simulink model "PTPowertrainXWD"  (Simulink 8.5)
settings: Solver=ode45  StartTime=0.0  StopTime=inf  RelTol=1e-3
libraries: CarMaker4SL x9, simulink x1
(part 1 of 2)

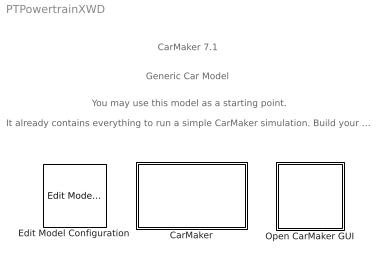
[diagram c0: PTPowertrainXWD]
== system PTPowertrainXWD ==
  note: Generic Car Model
  note: You may use this model as a starting point.
  note: It already contains everything to run a simple CarMaker simulation. Build your Simulink model around it.
  note: CarMaker 7.1
  CarMaker : Subsystem  TreatAsAtomicUnit=on
  Edit Model Configuration : CarMaker4SL/Edit Model Configuration
  Open CarMaker GUI : Subsystem  LoadFcn=if ~length(which('cmself')), cmenv; end

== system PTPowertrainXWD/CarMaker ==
  CM_FIRST : Subsystem
  CM_LAST : Subsystem
  DrivMan : Subsystem
  Ground : Ground
  IPG Vehicle : Subsystem  TreatAsAtomicUnit=on
  Terminator : Terminator
  VehicleControl : Subsystem
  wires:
  DrivMan/2(DrivMan.Out) -> VehicleControl/2(DrivMan.In)
  DrivMan/1(Sync_Out) -> VehicleControl/1(Sync_In)
  CM_FIRST/2(Env.Misc) -> DrivMan/2(Env.Misc)
  CM_FIRST/1(Sync_Out) -> DrivMan/1(Sync_In)
  CM_LAST/1(Sync_Out) -> Terminator/1
  Ground/1 -> CM_FIRST/1(Sync_In)
  IPG Vehicle/1(Sync_Out) -> CM_LAST/1(Sync_In)
  VehicleControl/1(Sync_Out) -> IPG Vehicle/1(Sync_In)
  VehicleControl/3(VhclCtrl.Steering) -> IPG Vehicle/3(VhclCtrl.Steering)
  VehicleControl/4(Vhcl.Wheel.In) -> IPG Vehicle/4(Vhcl.Wheel.In)
  VehicleControl/5(Vhcl.Misc) -> IPG Vehicle/5(Vhcl.Misc)
  VehicleControl/6(VhclCtrl.Brake) -> IPG Vehicle/6(VhclCtrl.Brake)
  VehicleControl/7(VhclCtrl.PT) -> IPG Vehicle/7(VhclCtrl.PT)
  VehicleControl/2(Vhcl.Model.Source) -> IPG Vehicle/2(Vhcl.Model.Source)

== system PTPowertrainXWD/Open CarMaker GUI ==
  S-Function : S-Function  FunctionName=cm_gui

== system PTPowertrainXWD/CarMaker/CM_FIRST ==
  Sync_In : Inport
  BusCreator1 : BusCreator  Inputs=8
  BusCreator2 : BusCreator  Inputs=6
  Demux1 : Demux  Outputs=14
  Environment : S-Function  FunctionName=CM_Sfun  Parameters='Environment'
  IoIn : S-Function  FunctionName=CM_Sfun  Parameters='IoIn'
  Terminator : Terminator
  Sync_Out : Outport
  Env.Misc : Outport  Port=2
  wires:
  BusCreator2/1 -> Terminator/1  "IF Environment (in)"
  BusCreator1/1 -> Env.Misc/1
  Demux1/14 -> BusCreator2/6  "Env sRoad"
  Demux1/13 -> BusCreator2/5  "Env PoI_GCS Elev"
  Demux1/12 -> BusCreator2/4  "Env PoI_GCS Lat"
  Demux1/11 -> BusCreator2/3  "Env PoI_GCS Long"
  Demux1/10 -> BusCreator2/2  "Env Time"
  Demux1/9 -> BusCreator2/1  "Env yDay"
  Demux1/8 -> BusCreator1/8  "Env WindVel_tot z"
  Demux1/7 -> BusCreator1/7  "Env WindVel_tot y"
  Demux1/6 -> BusCreator1/6  "Env WindVel_tot x"
  Demux1/5 -> BusCreator1/5  "Env SolarRadiation"
  Demux1/4 -> BusCreator1/4  "Env AirHumidity"
  Demux1/3 -> BusCreator1/3  "Env AirPressure"
  Demux1/2 -> BusCreator1/2  "Env AirDensity"
  Demux1/1 -> BusCreator1/1  "Env Temperature"
  Environment/2 -> Demux1/1
  Environment/1 -> Sync_Out/1
  IoIn/1 -> Environment/1
  Sync_In/1 -> IoIn/1

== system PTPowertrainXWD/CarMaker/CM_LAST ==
  Sync_In : Inport
  CM_User : S-Function  FunctionName=CM_Sfun  Parameters='CM_User'
  IoOut : S-Function  FunctionName=CM_Sfun  Parameters='IoOut'
  Sync_Out : Outport
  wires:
  IoOut/1 -> Sync_Out/1
  CM_User/1 -> IoOut/1
  Sync_In/1 -> CM_User/1

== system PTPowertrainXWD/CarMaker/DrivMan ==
  note: There's rarely a reason to override DrivMan signals. Use the VehicleControl interface for this purpose.
  Sync_In : Inport
  Env.Misc : Inport  Port=2
  BusCreator : BusCreator  Inputs=17
  Demux : Demux  Outputs=17
  DrivMan : S-Function  FunctionName=CM_Sfun  Parameters='DrivMan'
  Sync_Out : Outport
  DrivMan.Out : Outport  Port=2
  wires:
  Demux/17 -> BusCreator/17  "DrivMan Steering Trq"
  Demux/16 -> BusCreator/16  "DrivMan Steering AngAcc"
  Demux/15 -> BusCreator/15  "DrivMan Steering AngVel"
  Demux/14 -> BusCreator/14  "DrivMan Steering Ang"
  Demux/13 -> BusCreator/13  "DrivMan Gas"
  Demux/12 -> BusCreator/12  "DrivMan Clutch"
  Demux/11 -> BusCreator/11  "DrivMan BrakePark"
  Demux/10 -> BusCreator/10  "DrivMan Brake"
  Demux/9 -> BusCreator/9  "DrivMan GearNo"
  Demux/8 -> BusCreator/8  "DrivMan SelectorCtrl"
  Demux/7 -> BusCreator/7  "DrivMan UserSignal4"
  Demux/6 -> BusCreator/6  "DrivMan UserSignal3"
  Demux/5 -> BusCreator/5  "DrivMan UserSignal2"
  Demux/4 -> BusCreator/4  "DrivMan UserSignal1"
  Demux/3 -> BusCreator/3  "DrivMan UserSignal0"
  Demux/2 -> BusCreator/2  "DrivMan Key"
  Demux/1 -> BusCreator/1  "DrivMan SST"
  Env.Misc/1 -> DrivMan/2
  Sync_In/1 -> DrivMan/1
  DrivMan/1 -> Sync_Out/1
  BusCreator/1 -> DrivMan.Out/1
  DrivMan/2 -> Demux/1

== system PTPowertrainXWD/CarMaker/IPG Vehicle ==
  Sync_In : Inport
  Vhcl.Model.Source : Inport  Port=2
  VhclCtrl.Steering : Inport  Port=3
  Vhcl.Wheel.In : Inport  Port=4
  Vhcl.Misc : Inport  Port=5
  VhclCtrl.Brake : Inport  Port=6
  VhclCtrl.PT : Inport  Port=7
  Brake : Subsystem
  CarAndTrailer : Subsystem
  PowerTrain : Subsystem
  Stop Simulation : Stop
  VehicleSource_BuiltIn : simulink/Logic and Bit Operations/Compare To Constant  relop=~=  const=1  OutDataTypeStr=boolean  ZeroCross=off
  Sync_Out : Outport
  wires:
  VhclCtrl.PT/1 -> PowerTrain/3(VhclCtrl.PT)
  Brake/1(Sync_Out) -> PowerTrain/1(Sync_In)
  CarAndTrailer/1(Sync_Out) -> Brake/1(Sync_In)
  CarAndTrailer/2(Brake.IF.In) -> Brake/2(Brake.IF.In)
  VhclCtrl.Brake/1 -> Brake/3(VhclCtrl.Brake)
  PowerTrain/1(Sync_Out) -> Sync_Out/1
  Vhcl.Misc/1 -> CarAndTrailer/4(Vhcl.Misc)
  Vhcl.Wheel.In/1 -> CarAndTrailer/3(Vhcl.Wheel.In)
  VhclCtrl.Steering/1 -> CarAndTrailer/2(VhclCtrl.Steering)
  Sync_In/1 -> CarAndTrailer/1(Sync_In)
  Vhcl.Model.Source/1 -> VehicleSource_BuiltIn/1
  VehicleSource_BuiltIn/1 -> Stop Simulation/1
  Brake/2(Vhcl.Wheel.PT) -> PowerTrain/2(Vhcl.Wheel.PT)

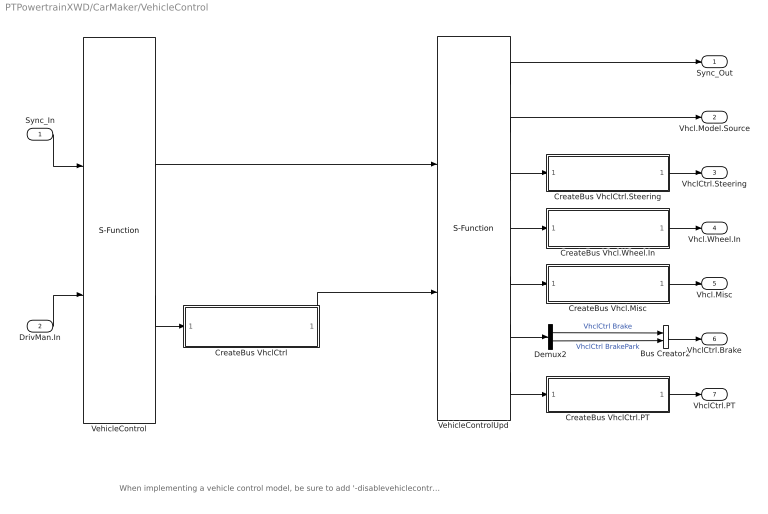
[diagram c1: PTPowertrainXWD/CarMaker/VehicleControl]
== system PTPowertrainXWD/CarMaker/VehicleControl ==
  note: When implementing a vehicle control model, be sure to add '-disablevehiclecontrol' to the command line arguments in the CarMaker Model Configuration block. Otherwise your model will possibly not see the original DrivMan signals on its inputs, but those of a currently activated C-coded vehicle control model instead.
  Sync_In : Inport
  DrivMan.In : Inport  Port=2
  Bus Creator2 : BusCreator  Inputs=2
  CreateBus Vhcl.Misc : Subsystem
  CreateBus Vhcl.Wheel.In : Subsystem
  CreateBus VhclCtrl : Subsystem
  CreateBus VhclCtrl.PT : Subsystem
  CreateBus VhclCtrl.Steering : Subsystem
  Demux2 : Demux  Outputs=2
  VehicleControl : S-Function  FunctionName=CM_Sfun  Parameters='VehicleControl'
  VehicleControlUpd : S-Function  FunctionName=CM_Sfun  Parameters='VehicleControlUpd'
  Sync_Out : Outport
  Vhcl.Model.Source : Outport  Port=2
  VhclCtrl.Steering : Outport  Port=3
  Vhcl.Wheel.In : Outport  Port=4
  Vhcl.Misc : Outport  Port=5
  VhclCtrl.Brake : Outport  Port=6
  VhclCtrl.PT : Outport  Port=7
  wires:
  CreateBus VhclCtrl/1(Out) -> VehicleControlUpd/2
  VehicleControl/2 -> CreateBus VhclCtrl/1(In)
  VehicleControlUpd/2 -> Vhcl.Model.Source/1
  VehicleControlUpd/4 -> CreateBus Vhcl.Wheel.In/1(In1)
  VehicleControlUpd/5 -> CreateBus Vhcl.Misc/1(In1)
  VehicleControlUpd/6 -> Demux2/1
  VehicleControlUpd/7 -> CreateBus VhclCtrl.PT/1(In1)
  VehicleControlUpd/3 -> CreateBus VhclCtrl.Steering/1(In1)
  CreateBus Vhcl.Misc/1(Out1) -> Vhcl.Misc/1
  CreateBus Vhcl.Wheel.In/1(Out1) -> Vhcl.Wheel.In/1
  DrivMan.In/1 -> VehicleControl/2
  VehicleControl/1 -> VehicleControlUpd/1
  Sync_In/1 -> VehicleControl/1
  CreateBus VhclCtrl.PT/1(Out1) -> VhclCtrl.PT/1
  Bus Creator2/1 -> VhclCtrl.Brake/1
  CreateBus VhclCtrl.Steering/1(Out1) -> VhclCtrl.Steering/1
  VehicleControlUpd/1 -> Sync_Out/1
  Demux2/2 -> Bus Creator2/2  "VhclCtrl BrakePark"
  Demux2/1 -> Bus Creator2/1  "VhclCtrl Brake"

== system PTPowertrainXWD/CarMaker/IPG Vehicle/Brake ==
  note: When replacing the entire braking system, be sure to add '-disablebrake' to the command line arguments in the CarMaker Model Configuration block.
  Sync_In : Inport
  Brake.IF.In : Inport  Port=2
  VhclCtrl.Brake : Inport  Port=3
  Brake : S-Function  FunctionName=CM_Sfun  Parameters='Brake'
  BrakeUpd : S-Function  FunctionName=CM_Sfun  Parameters='BrakeUpd'
  BusCreator1 : BusCreator  Inputs=16
  CreateBus Vhcl.Wheel.PT : Subsystem
  Demux : Demux  Outputs=16
  Sync_Out : Outport
  Vhcl.Wheel.PT : Outport  Port=2
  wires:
  Demux/16 -> BusCreator1/16  "Brake IF Trq_DriveSrc_trg d3"
  Demux/15 -> BusCreator1/15  "Brake IF Trq_DriveSrc_trg d2"
  Demux/14 -> BusCreator1/14  "Brake IF Trq_DriveSrc_trg d1"
  Demux/13 -> BusCreator1/13  "Brake IF Trq_DriveSrc_trg d0"
  Demux/12 -> BusCreator1/12  "Brake IF Trq_Reg_trg RR"
  Demux/11 -> BusCreator1/11  "Brake IF Trq_Reg_trg RL"
  Demux/10 -> BusCreator1/10  "Brake IF Trq_Reg_trg FR"
  Demux/9 -> BusCreator1/9  "Brake IF Trq_Reg_trg FL"
  Demux/8 -> BusCreator1/8  "Brake IF Trq_PB RR"
  Demux/7 -> BusCreator1/7  "Brake IF Trq_PB RL"
  Demux/6 -> BusCreator1/6  "Brake IF Trq_PB FR"
  Demux/5 -> BusCreator1/5  "Brake IF Trq_PB FL"
  Demux/4 -> BusCreator1/4  "Brake IF Trq_WB RR"
  Demux/3 -> BusCreator1/3  "Brake IF Trq_WB RL"
  Demux/2 -> BusCreator1/2  "Brake IF Trq_WB FR"
  Demux/1 -> BusCreator1/1  "Brake IF Trq_WB FL"
  Brake/2 -> Demux/1
  BusCreator1/1 -> BrakeUpd/2
  BrakeUpd/1 -> Sync_Out/1
  Brake/1 -> BrakeUpd/1  "Sync"
  Brake.IF.In/1 -> Brake/2
  VhclCtrl.Brake/1 -> Brake/3
  Sync_In/1 -> Brake/1
  BrakeUpd/2 -> CreateBus Vhcl.Wheel.PT/1(In)
  CreateBus Vhcl.Wheel.PT/1(Out) -> Vhcl.Wheel.PT/1

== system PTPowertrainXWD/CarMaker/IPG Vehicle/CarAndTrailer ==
  Sync_In : Inport
  VhclCtrl.Steering : Inport  Port=2
  Vhcl.Wheel.In : Inport  Port=3
  Vhcl.Misc : Inport  Port=4
  CarAndTrailerUpd : Subsystem
  Forces : Subsystem
  Ground : Ground
  Kinematics : Subsystem
  Kinetics : Subsystem
  Steering : Subsystem
  Terminator : Terminator
  Terminator1 : Terminator
  Trailer : Subsystem
  Sync_Out : Outport
  Brake.IF.In : Outport  Port=2
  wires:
  Trailer/9(Car.Hitch.FrcTrq) -> CarAndTrailerUpd/9(Car.Hitch.FrcTrq)
  Trailer/8(Vhcl.Wheel.RR) -> CarAndTrailerUpd/8(Vhcl.Wheel.RR)
  Trailer/7(Vhcl.Wheel.RL) -> CarAndTrailerUpd/7(Vhcl.Wheel.RL)
  Trailer/6(Vhcl.Wheel.FR) -> CarAndTrailerUpd/6(Vhcl.Wheel.FR)
  Trailer/5(Vhcl.Wheel.FL) -> CarAndTrailerUpd/5(Vhcl.Wheel.FL)
  Trailer/4(Vhcl.PoI) -> CarAndTrailerUpd/4(Vhcl.PoI)
  Trailer/3(Vhcl.Motion) -> CarAndTrailerUpd/3(Vhcl.Motion)
  Trailer/2(Vhcl.Steering) -> CarAndTrailerUpd/2(Vhcl.Steering)
  Trailer/1(Sync_Out) -> CarAndTrailerUpd/1(Sync_In)
  CarAndTrailerUpd/2(Brake.IF.In) -> Brake.IF.In/1
  CarAndTrailerUpd/1(Sync_Out) -> Sync_Out/1
  Vhcl.Misc/1 -> Terminator1/1
  Vhcl.Wheel.In/1 -> Terminator/1
  Kinetics/6(WheelCarrier.Misc) -> Trailer/6(WheelCarrier.Misc)
  Kinetics/5(Car.Trq_T2W) -> Trailer/5(Car.Trq_T2W)
  Steering/2(Steer.IF) -> Kinematics/2(Steer.IF)
  Kinetics/4(Car.Fr1) -> Trailer/4(Car.Fr1)
  Kinetics/3(Car.Hitch) -> Trailer/3(Car.Hitch)
  Kinetics/2(Trailer.Load) -> Trailer/2(Trailer.Load)
  VhclCtrl.Steering/1 -> Steering/2(VhclCtrl.Steering)
  Sync_In/1 -> Steering/1(Sync_In)
  Steering/1(Sync_Out) -> Kinematics/1(Sync_In)
  Kinetics/1(Sync_Out) -> Trailer/1(Sync_In)
  Ground/1 -> CarAndTrailerUpd/10(Vhcl.Fr1A)
  Forces/11(FStabi) -> Kinetics/11(FStabi)
  Forces/10(FDamp) -> Kinetics/10(FDamp)
  Forces/9(FSpring) -> Kinetics/9(FSpring)
  Forces/8(TireRR_Out) -> Kinetics/8(TireRR.Out)
  Forces/7(TireRL_Out) -> Kinetics/7(TireRL.Out)
  Forces/6(TireFR_Out) -> Kinetics/6(TireFR.Out)
  Forces/5(TireFL_Out) -> Kinetics/5(TireFL.Out)
  Forces/4(Car.Load) -> Kinetics/4(Car.Load)
  Forces/2(Car.Virtual) -> Kinetics/2(Car.Virtual)
  Kinematics/6(lSpring) -> Forces/6(lSpring)
  Kinematics/7(vDamp) -> Forces/7(vDamp)
  Forces/3(Car.Aero) -> Kinetics/3(Car.Aero)
  Forces/1(Sync_Out) -> Kinetics/1(Sync_In)
  Kinematics/5(TireRR_In) -> Forces/5(TireRR_In)
  Kinematics/4(TireRL_In) -> Forces/4(TireRL_In)
  Kinematics/3(TireFR_In) -> Forces/3(TireFR_In)
  Kinematics/2(TireFL_In) -> Forces/2(TireFL_In)
  Kinematics/1(Sync_Out) -> Forces/1(Sync_In)
  Kinematics/8(lStabi) -> Forces/8(lStabi)
  Forces/12(FBuf) -> Kinetics/12(FBuf)
  Kinematics/9(lBuf) -> Forces/9(lBuf)

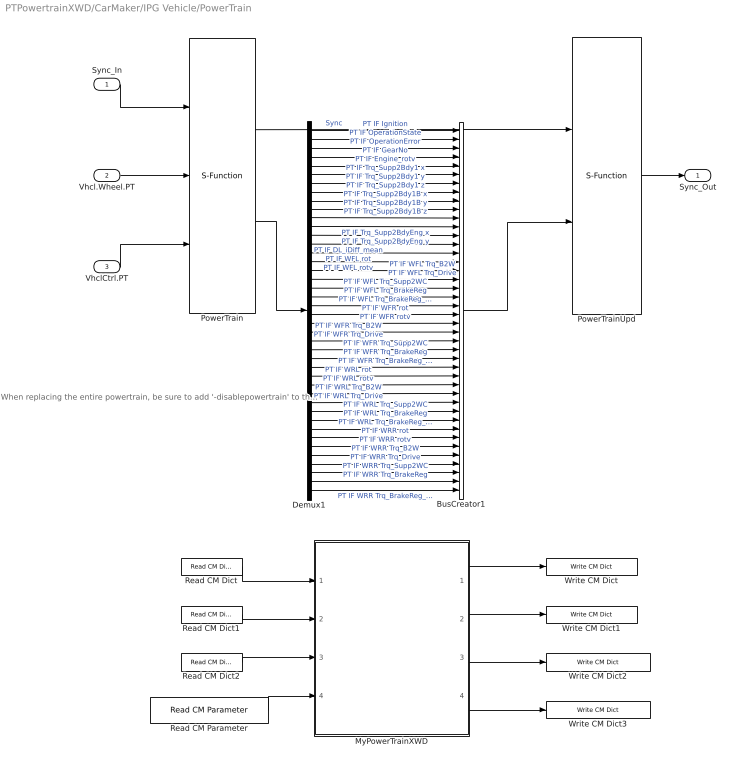
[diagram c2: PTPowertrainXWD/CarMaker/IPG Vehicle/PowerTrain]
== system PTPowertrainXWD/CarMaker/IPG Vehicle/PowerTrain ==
  note: When replacing the entire powertrain, be sure to add '-disablepowertrain' to the command line arguments in the CarMaker Model Configuration block.
  Sync_In : Inport
  Vhcl.Wheel.PT : Inport  Port=2
  VhclCtrl.PT : Inport  Port=3
  BusCreator1 : BusCreator  Inputs=42
  Demux1 : Demux  Outputs=42
  MyPowerTrainXWD : Subsystem
  PowerTrain : S-Function  FunctionName=CM_Sfun  Parameters='PowerTrain'
  PowerTrainUpd : S-Function  FunctionName=CM_Sfun  Parameters='PowerTrainUpd'
  Read CM Dict : CarMaker4SL/Read CM Dict  xname=PT.WFL.rotv  xsync=off
  Read CM Dict1 : CarMaker4SL/Read CM Dict  xname=PT.WFR.rotv  xsync=off
  Read CM Dict2 : CarMaker4SL/Read CM Dict  xname=VC.Gas  xsync=off
  Read CM Parameter : CarMaker4SL/Read CM Parameter  xfile=Vehicle  xkey=PowerTrain.DL.iDiff_mean  xnout=1  xdefaults=0  xmuxed=on
  Write CM Dict : CarMaker4SL/Write CM Dict  xname=PT.WFL.Trq_Drive  xsync=off
  Write CM Dict1 : CarMaker4SL/Write CM Dict  xname=PT.WFR.Trq_Drive  xsync=off
  Write CM Dict2 : CarMaker4SL/Write CM Dict  xname=PT.WFL.Trq_Supp2WC  xsync=off
  Write CM Dict3 : CarMaker4SL/Write CM Dict  xname=PT.WFL.Trq_Supp2WC  xsync=off
  Sync_Out : Outport
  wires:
  BusCreator1/1 -> PowerTrainUpd/2
  Demux1/42 -> BusCreator1/42  "PT IF WRR Trq_BrakeReg_max"
  Demux1/41 -> BusCreator1/41  "PT IF WRR Trq_BrakeReg"
  Demux1/40 -> BusCreator1/40  "PT IF WRR Trq_Supp2WC"
  Demux1/39 -> BusCreator1/39  "PT IF WRR Trq_Drive"
  Demux1/38 -> BusCreator1/38  "PT IF WRR Trq_B2W"
  Demux1/37 -> BusCreator1/37  "PT IF WRR rotv"
  Demux1/36 -> BusCreator1/36  "PT IF WRR rot"
  Demux1/35 -> BusCreator1/35  "PT IF WRL Trq_BrakeReg_max"
  Demux1/34 -> BusCreator1/34  "PT IF WRL Trq_BrakeReg"
  Demux1/33 -> BusCreator1/33  "PT IF WRL Trq_Supp2WC"
  Demux1/32 -> BusCreator1/32  "PT IF WRL Trq_Drive"
  Demux1/31 -> BusCreator1/31  "PT IF WRL Trq_B2W"
  Demux1/30 -> BusCreator1/30  "PT IF WRL rotv"
  Demux1/29 -> BusCreator1/29  "PT IF WRL rot"
  Demux1/28 -> BusCreator1/28  "PT IF WFR Trq_BrakeReg_max"
  Demux1/27 -> BusCreator1/27  "PT IF WFR Trq_BrakeReg"
  Demux1/26 -> BusCreator1/26  "PT IF WFR Trq_Supp2WC"
  Demux1/25 -> BusCreator1/25  "PT IF WFR Trq_Drive"
  Demux1/24 -> BusCreator1/24  "PT IF WFR Trq_B2W"
  Demux1/23 -> BusCreator1/23  "PT IF WFR rotv"
  Demux1/22 -> BusCreator1/22  "PT IF WFR rot"
  Demux1/21 -> BusCreator1/21  "PT IF WFL Trq_BrakeReg_max"
  Demux1/20 -> BusCreator1/20  "PT IF WFL Trq_BrakeReg"
  Demux1/19 -> BusCreator1/19  "PT IF WFL Trq_Supp2WC"
  Demux1/18 -> BusCreator1/18  "PT IF WFL Trq_Drive"
  Demux1/17 -> BusCreator1/17  "PT IF WFL Trq_B2W"
  Demux1/16 -> BusCreator1/16  "PT IF WFL rotv"
  Demux1/15 -> BusCreator1/15  "PT IF WFL rot"
  Demux1/14 -> BusCreator1/14  "PT IF DL_iDiff_mean"
  Demux1/13 -> BusCreator1/13  "PT IF Trq_Supp2BdyEng y"
  Demux1/12 -> BusCreator1/12  "PT IF Trq_Supp2BdyEng x"
  Demux1/11 -> BusCreator1/11  "PT IF Trq_Supp2Bdy1B z"
  Demux1/10 -> BusCreator1/10  "PT IF Trq_Supp2Bdy1B y"
  Demux1/9 -> BusCreator1/9  "PT IF Trq_Supp2Bdy1B x"
  Demux1/8 -> BusCreator1/8  "PT IF Trq_Supp2Bdy1 z"
  Demux1/7 -> BusCreator1/7  "PT IF Trq_Supp2Bdy1 y"
  Demux1/6 -> BusCreator1/6  "PT IF Trq_Supp2Bdy1 x"
  Demux1/5 -> BusCreator1/5  "PT IF Engine_rotv"
  Demux1/4 -> BusCreator1/4  "PT IF GearNo"
  Demux1/3 -> BusCreator1/3  "PT IF OperationError"
  Demux1/2 -> BusCreator1/2  "PT IF OperationState"
  Demux1/1 -> BusCreator1/1  "PT IF Ignition"
  Sync_In/1 -> PowerTrain/1
  PowerTrain/2 -> Demux1/1
  PowerTrainUpd/1 -> Sync_Out/1
  PowerTrain/1 -> PowerTrainUpd/1  "Sync"
  VhclCtrl.PT/1 -> PowerTrain/3
  Vhcl.Wheel.PT/1 -> PowerTrain/2
  MyPowerTrainXWD/1(PT.WFL.Trq_Drive) -> Write CM Dict/1
  MyPowerTrainXWD/2(PT.WFR.Trq_Drive) -> Write CM Dict1/1
  MyPowerTrainXWD/3(PT.WFL.Trq_Supp2WC) -> Write CM Dict2/1
  MyPowerTrainXWD/4(PT.WFR.Trq_Supp2WC) -> Write CM Dict3/1
  Read CM Dict/1 -> MyPowerTrainXWD/1(PT.WFL.rotv)
  Read CM Dict1/1 -> MyPowerTrainXWD/2(PT.WFR.rotv)
  Read CM Dict2/1 -> MyPowerTrainXWD/3(Gas)
  Read CM Parameter/1 -> MyPowerTrainXWD/4(iDiff_mean)

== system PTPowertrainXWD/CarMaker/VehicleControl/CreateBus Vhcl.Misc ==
  In1 : Inport
  BusCreator : BusCreator  Inputs=11
  Demux : Demux  Outputs=11
  Out1 : Outport
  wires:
  Demux/11 -> BusCreator/11  "Vhcl Wind_vel_0 z"
  Demux/10 -> BusCreator/10  "Vhcl Wind_vel_0 y"
  Demux/9 -> BusCreator/9  "Vhcl Wind_vel_0 x"
  Demux/8 -> BusCreator/8  "Vhcl Trq_DL2BdyEng y"
  Demux/7 -> BusCreator/7  "Vhcl Trq_DL2BdyEng x"
  Demux/6 -> BusCreator/6  "Vhcl Trq_DL2Bdy1B z"
  Demux/5 -> BusCreator/5  "Vhcl Trq_DL2Bdy1B y"
  Demux/4 -> BusCreator/4  "Vhcl Trq_DL2Bdy1B x"
  Demux/3 -> BusCreator/3  "Vhcl Trq_DL2Bdy1 z"
  Demux/2 -> BusCreator/2  "Vhcl Trq_DL2Bdy1 y"
  Demux/1 -> BusCreator/1  "Vhcl Trq_DL2Bdy1 x"
  In1/1 -> Demux/1
  BusCreator/1 -> Out1/1

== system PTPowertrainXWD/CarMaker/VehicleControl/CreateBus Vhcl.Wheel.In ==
  In1 : Inport
  Bus Creator1 : BusCreator  Inputs=12
  Demux1 : Demux  Outputs=12
  Out1 : Outport
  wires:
  Demux1/12 -> Bus Creator1/12  "Vhcl Wheel RR rotv"
  Demux1/11 -> Bus Creator1/11  "Vhcl Wheel RR Trq_DL2WC"
  Demux1/10 -> Bus Creator1/10  "Vhcl Wheel RR Trq_B2WC"
  Demux1/9 -> Bus Creator1/9  "Vhcl Wheel RL rotv"
  Demux1/8 -> Bus Creator1/8  "Vhcl Wheel RL Trq_DL2WC"
  Demux1/7 -> Bus Creator1/7  "Vhcl Wheel RL Trq_B2WC"
  Demux1/6 -> Bus Creator1/6  "Vhcl Wheel FR rotv"
  Demux1/5 -> Bus Creator1/5  "Vhcl Wheel FR Trq_DL2WC"
  Demux1/4 -> Bus Creator1/4  "Vhcl Wheel FR Trq_B2WC"
  Demux1/3 -> Bus Creator1/3  "Vhcl Wheel FL rotv"
  In1/1 -> Demux1/1
  Bus Creator1/1 -> Out1/1
  Demux1/2 -> Bus Creator1/2  "Vhcl Wheel FL Trq_DL2WC"
  Demux1/1 -> Bus Creator1/1  "Vhcl Wheel FL Trq_B2WC"

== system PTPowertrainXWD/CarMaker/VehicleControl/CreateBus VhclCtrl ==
  In : Inport
  BusCreator : BusCreator  Inputs=29
  Demux : Demux  Outputs=29
  Out : Outport
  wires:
  In/1 -> Demux/1
  BusCreator/1 -> Out/1
  Demux/1 -> BusCreator/1  "VhclCtrl SST"
  Demux/2 -> BusCreator/2  "VhclCtrl Key"
  Demux/3 -> BusCreator/3  "VhclCtrl UserSignal0"
  Demux/4 -> BusCreator/4  "VhclCtrl UserSignal1"
  Demux/5 -> BusCreator/5  "VhclCtrl UserSignal2"
  Demux/6 -> BusCreator/6  "VhclCtrl UserSignal3"
  Demux/7 -> BusCreator/7  "VhclCtrl UserSignal4"
  Demux/8 -> BusCreator/8  "VhclCtrl GearNo"
  Demux/9 -> BusCreator/9  "VhclCtrl SelectorCtrl"
  Demux/10 -> BusCreator/10  "VhclCtrl Brake"
  Demux/11 -> BusCreator/11  "VhclCtrl BrakePark"
  Demux/12 -> BusCreator/12  "VhclCtrl Clutch"
  Demux/13 -> BusCreator/13  "VhclCtrl Gas"
  Demux/14 -> BusCreator/14  "VhclCtrl Steering Ang"
  Demux/15 -> BusCreator/15  "VhclCtrl Steering AngVel"
  Demux/16 -> BusCreator/16  "VhclCtrl Steering AngAcc"
  Demux/17 -> BusCreator/17  "VhclCtrl Steering Trq"
  Demux/18 -> BusCreator/18  "VhclCtrl Lights LowBeam"
  Demux/19 -> BusCreator/19  "VhclCtrl Lights HighBeam"
  Demux/20 -> BusCreator/20  "VhclCtrl Lights Daytime"
  Demux/21 -> BusCreator/21  "VhclCtrl Lights ParkL"
  Demux/22 -> BusCreator/22  "VhclCtrl Lights ParkR"
  Demux/23 -> BusCreator/23  "VhclCtrl Lights IndL"
  Demux/24 -> BusCreator/24  "VhclCtrl Lights IndR"
  Demux/25 -> BusCreator/25  "VhclCtrl Lights FogFrontL"
  Demux/26 -> BusCreator/26  "VhclCtrl Lights FogFrontR"
  Demux/27 -> BusCreator/27  "VhclCtrl Lights FogRear"
  Demux/28 -> BusCreator/28  "VhclCtrl Lights Brake"
  Demux/29 -> BusCreator/29  "VhclCtrl Lights Reverse"

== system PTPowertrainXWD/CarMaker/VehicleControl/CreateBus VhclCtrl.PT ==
  In1 : Inport
  BusCreator1 : BusCreator  Inputs=12
  Demux1 : Demux  Outputs=12
  Out1 : Outport
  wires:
  Demux1/12 -> BusCreator1/12  "VhclCtrl Brake"
  Demux1/11 -> BusCreator1/11  "VhclCtrl Gas"
  Demux1/10 -> BusCreator1/10  "VhclCtrl Clutch"
  Demux1/9 -> BusCreator1/9  "VhclCtrl SelectorCtrl"
  Demux1/8 -> BusCreator1/8  "VhclCtrl GearNo"
  Demux1/7 -> BusCreator1/7  "VhclCtrl UserSignal4"
  Demux1/6 -> BusCreator1/6  "VhclCtrl UserSignal3"
  Demux1/5 -> BusCreator1/5  "VhclCtrl UserSignal2"
  Demux1/4 -> BusCreator1/4  "VhclCtrl UserSignal1"
  Demux1/3 -> BusCreator1/3  "VhclCtrl UserSignal0"
  Demux1/2 -> BusCreator1/2  "VhclCtrl Key"
  Demux1/1 -> BusCreator1/1  "VhclCtrl SST"
  In1/1 -> Demux1/1
  BusCreator1/1 -> Out1/1

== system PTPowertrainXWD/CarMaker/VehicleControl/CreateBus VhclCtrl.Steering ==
  In1 : Inport
  Bus Creator : BusCreator  Inputs=5
  Demux : Demux  Outputs=5
  Out1 : Outport
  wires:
  In1/1 -> Demux/1
  Bus Creator/1 -> Out1/1
  Demux/1 -> Bus Creator/1  "VhclCtrl Steering Ang"
  Demux/5 -> Bus Creator/5  "VhclCtrl Steering SteerByTrq"
  Demux/3 -> Bus Creator/3  "VhclCtrl Steering AngAcc"
  Demux/2 -> Bus Creator/2  "VhclCtrl Steering AngVel"
  Demux/4 -> Bus Creator/4  "VhclCtrl Steering Trq"

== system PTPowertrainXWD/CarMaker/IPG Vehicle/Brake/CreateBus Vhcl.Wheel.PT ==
  In : Inport
  BusCreator1 : BusCreator  Inputs=20
  Demux1 : Demux  Outputs=20
  Out : Outport
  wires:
  Demux1/20 -> BusCreator1/20  "Vhcl Trq_DriveSrc_trg d3"
  Demux1/19 -> BusCreator1/19  "Vhcl Trq_DriveSrc_trg d2"
  Demux1/18 -> BusCreator1/18  "Vhcl Trq_DriveSrc_trg d1"
  Demux1/17 -> BusCreator1/17  "Vhcl Trq_DriveSrc_trg d0"
  Demux1/16 -> BusCreator1/16  "Vhcl Wheel RR WhlBearing"
  Demux1/15 -> BusCreator1/15  "Vhcl Wheel RR Trq_T2W"
  Demux1/14 -> BusCreator1/14  "Vhcl Wheel RR Trq_BrakeReg_trg"
  Demux1/13 -> BusCreator1/13  "Vhcl Wheel RR Trq_Brake"
  Demux1/12 -> BusCreator1/12  "Vhcl Wheel RL WhlBearing"
  Demux1/11 -> BusCreator1/11  "Vhcl Wheel RL Trq_T2W"
  Demux1/10 -> BusCreator1/10  "Vhcl Wheel RL Trq_BrakeReg_trg"
  Demux1/9 -> BusCreator1/9  "Vhcl Wheel RL Trq_Brake"
  Demux1/8 -> BusCreator1/8  "Vhcl Wheel FR WhlBearing"
  Demux1/7 -> BusCreator1/7  "Vhcl Wheel FR Trq_T2W"
  Demux1/6 -> BusCreator1/6  "Vhcl Wheel FR Trq_BrakeReg_trg"
  Demux1/5 -> BusCreator1/5  "Vhcl Wheel FR Trq_Brake"
  Demux1/4 -> BusCreator1/4  "Vhcl Wheel FL WhlBearing"
  Demux1/3 -> BusCreator1/3  "Vhcl Wheel FL Trq_T2W"
  Demux1/2 -> BusCreator1/2  "Vhcl Wheel FL Trq_BrakeReg_trg"
  Demux1/1 -> BusCreator1/1  "Vhcl Wheel FL Trq_Brake"
  BusCreator1/1 -> Out/1
  In/1 -> Demux1/1

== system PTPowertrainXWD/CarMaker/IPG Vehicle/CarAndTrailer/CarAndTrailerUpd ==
  Sync_In : Inport
  Vhcl.Steering : Inport  Port=2
  Vhcl.Motion : Inport  Port=3
  Vhcl.PoI : Inport  Port=4
  Vhcl.Wheel.FL : Inport  Port=5
  Vhcl.Wheel.FR : Inport  Port=6
  Vhcl.Wheel.RL : Inport  Port=7
  Vhcl.Wheel.RR : Inport  Port=8
  Car.Hitch.FrcTrq : Inport  Port=9
  Vhcl.Fr1A : Inport  Port=10
  CarAndTrailerUpd : S-Function  FunctionName=CM_Sfun  Parameters='CarAndTrUpd'
  CreateBus Brake.IF.In : Subsystem
  Sync_Out : Outport
  Brake.IF.In : Outport  Port=2
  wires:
  Vhcl.Fr1A/1 -> CarAndTrailerUpd/10  "user vehicle only"
  Vhcl.Steering/1 -> CarAndTrailerUpd/2
  Vhcl.Motion/1 -> CarAndTrailerUpd/3
  Vhcl.PoI/1 -> CarAndTrailerUpd/4
  Vhcl.Wheel.FL/1 -> CarAndTrailerUpd/5
  Vhcl.Wheel.FR/1 -> CarAndTrailerUpd/6
  Car.Hitch.FrcTrq/1 -> CarAndTrailerUpd/9
  Vhcl.Wheel.RR/1 -> CarAndTrailerUpd/8
  Vhcl.Wheel.RL/1 -> CarAndTrailerUpd/7
  CarAndTrailerUpd/2 -> CreateBus Brake.IF.In/1(In)
  CreateBus Brake.IF.In/1(Out) -> Brake.IF.In/1
  CarAndTrailerUpd/1 -> Sync_Out/1
  Sync_In/1 -> CarAndTrailerUpd/1

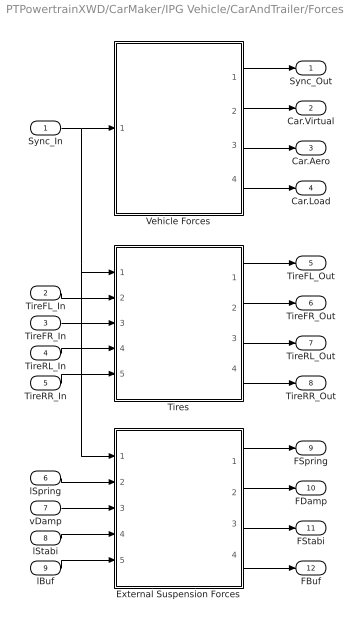
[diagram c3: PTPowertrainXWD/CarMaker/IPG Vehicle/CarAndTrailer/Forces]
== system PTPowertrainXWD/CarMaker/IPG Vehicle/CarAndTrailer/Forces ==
  Sync_In : Inport
  TireFL_In : Inport  Port=2
  TireFR_In : Inport  Port=3
  TireRL_In : Inport  Port=4
  TireRR_In : Inport  Port=5
  lSpring : Inport  Port=6
  vDamp : Inport  Port=7
  lStabi : Inport  Port=8
  lBuf : Inport  Port=9
  External Suspension Forces : Subsystem
  Tires : Subsystem
  Vehicle Forces : Subsystem
  Sync_Out : Outport
  Car.Virtual : Outport  Port=2
  Car.Aero : Outport  Port=3
  Car.Load : Outport  Port=4
  TireFL_Out : Outport  Port=5
  TireFR_Out : Outport  Port=6
  TireRL_Out : Outport  Port=7
  TireRR_Out : Outport  Port=8
  FSpring : Outport  Port=9
  FDamp : Outport  Port=10
  FStabi : Outport  Port=11
  FBuf : Outport  Port=12
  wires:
  lBuf/1 -> External Suspension Forces/5(lBuf)
  lStabi/1 -> External Suspension Forces/4(lStabi)
  vDamp/1 -> External Suspension Forces/3(vDamp)
  Tires/4(TireRR_Out) -> TireRR_Out/1
  Tires/3(TireRL_Out) -> TireRL_Out/1
  Tires/2(TireFR_Out) -> TireFR_Out/1
  Tires/1(TireFL_Out) -> TireFL_Out/1
  TireRR_In/1 -> Tires/5(TireRR_In)
  TireRL_In/1 -> Tires/4(TireRL_In)
  TireFR_In/1 -> Tires/3(TireFR_In)
  TireFL_In/1 -> Tires/2(TireFL_In)
  External Suspension Forces/4(FBuf) -> FBuf/1
  Sync_In/1 -> External Suspension Forces/1(Sync_In), Tires/1(Sync_In), Vehicle Forces/1(Sync_In)
  Vehicle Forces/1(Sync_Out) -> Sync_Out/1
  Vehicle Forces/2(Car.Virtual) -> Car.Virtual/1
  Vehicle Forces/3(Car.Aero) -> Car.Aero/1
  Vehicle Forces/4(Car.Load) -> Car.Load/1
  lSpring/1 -> External Suspension Forces/2(lSpring)
  External Suspension Forces/2(FDamp) -> FDamp/1
  External Suspension Forces/3(FStabi) -> FStabi/1
  External Suspension Forces/1(FSpring) -> FSpring/1

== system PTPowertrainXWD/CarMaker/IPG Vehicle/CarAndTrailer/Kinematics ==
  Sync_In : Inport
  Steer.IF : Inport  Port=2
  Kinematics : S-Function  FunctionName=CM_Sfun  Parameters='Kinematics'
  Sync_Out : Outport
  TireFL_In : Outport  Port=2
  TireFR_In : Outport  Port=3
  TireRL_In : Outport  Port=4
  TireRR_In : Outport  Port=5
  lSpring : Outport  Port=6
  vDamp : Outport  Port=7
  lStabi : Outport  Port=8
  lBuf : Outport  Port=9
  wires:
  Kinematics/9 -> lBuf/1
  Kinematics/8 -> lStabi/1
  Kinematics/2 -> TireFL_In/1
  Kinematics/3 -> TireFR_In/1
  Kinematics/4 -> TireRL_In/1
  Kinematics/5 -> TireRR_In/1
  Kinematics/6 -> lSpring/1
  Kinematics/7 -> vDamp/1
  Sync_In/1 -> Kinematics/1
  Kinematics/1 -> Sync_Out/1
  Steer.IF/1 -> Kinematics/2

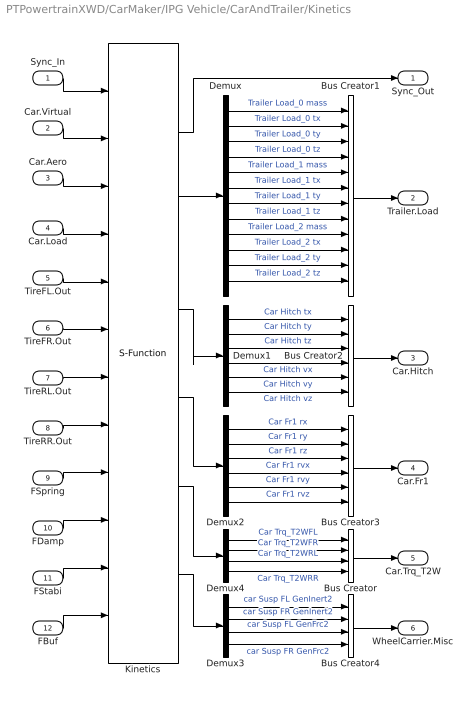
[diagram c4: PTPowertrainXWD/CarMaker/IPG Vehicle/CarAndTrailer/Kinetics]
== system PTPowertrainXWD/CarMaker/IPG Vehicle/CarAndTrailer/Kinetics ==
  Sync_In : Inport
  Car.Virtual : Inport  Port=2
  Car.Aero : Inport  Port=3
  Car.Load : Inport  Port=4
  TireFL.Out : Inport  Port=5
  TireFR.Out : Inport  Port=6
  TireRL.Out : Inport  Port=7
  TireRR.Out : Inport  Port=8
  FSpring : Inport  Port=9
  FDamp : Inport  Port=10
  FStabi : Inport  Port=11
  FBuf : Inport  Port=12
  Bus Creator : BusCreator
  Bus Creator1 : BusCreator  Inputs=12
  Bus Creator2 : BusCreator  Inputs=6
  Bus Creator3 : BusCreator  Inputs=6
  Bus Creator4 : BusCreator
  Demux : Demux  Outputs=12
  Demux1 : Demux  Outputs=6
  Demux2 : Demux  Outputs=6
  Demux3 : Demux
  Demux4 : Demux
  Kinetics : S-Function  FunctionName=CM_Sfun  Parameters='Kinetics'
  Sync_Out : Outport
  Trailer.Load : Outport  Port=2
  Car.Hitch : Outport  Port=3
  Car.Fr1 : Outport  Port=4
  Car.Trq_T2W : Outport  Port=5
  WheelCarrier.Misc : Outport  Port=6
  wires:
  FBuf/1 -> Kinetics/12
  Sync_In/1 -> Kinetics/1
  Kinetics/1 -> Sync_Out/1
  Car.Aero/1 -> Kinetics/3
  Car.Virtual/1 -> Kinetics/2
  Bus Creator1/1 -> Trailer.Load/1
  Demux/1 -> Bus Creator1/1  "Trailer Load_0 mass"
  Demux/2 -> Bus Creator1/2  "Trailer Load_0 tx"
  Demux/3 -> Bus Creator1/3  "Trailer Load_0 ty"
  Demux/4 -> Bus Creator1/4  "Trailer Load_0 tz"
  Kinetics/2 -> Demux/1
  Demux/5 -> Bus Creator1/5  "Trailer Load_1 mass"
  Demux/6 -> Bus Creator1/6  "Trailer Load_1 tx"
  Demux/7 -> Bus Creator1/7  "Trailer Load_1 ty"
  Demux/8 -> Bus Creator1/8  "Trailer Load_1 tz"
  Demux/9 -> Bus Creator1/9  "Trailer Load_2 mass"
  Demux/10 -> Bus Creator1/10  "Trailer Load_2 tx"
  Demux/11 -> Bus Creator1/11  "Trailer Load_2 ty"
  Demux/12 -> Bus Creator1/12  "Trailer Load_2 tz"
  Demux1/1 -> Bus Creator2/1  "Car Hitch tx"
  Demux1/2 -> Bus Creator2/2  "Car Hitch ty"
  Demux1/3 -> Bus Creator2/3  "Car Hitch tz"
  Demux1/4 -> Bus Creator2/4  "Car Hitch vx"
  Demux1/5 -> Bus Creator2/5  "Car Hitch vy"
  Demux1/6 -> Bus Creator2/6  "Car Hitch vz"
  Kinetics/3 -> Demux1/1
  Bus Creator2/1 -> Car.Hitch/1
  Demux2/1 -> Bus Creator3/1  "Car Fr1 rx"
  Demux2/2 -> Bus Creator3/2  "Car Fr1 ry"
  Demux2/3 -> Bus Creator3/3  "Car Fr1 rz"
  Demux2/4 -> Bus Creator3/4  "Car Fr1 rvx"
  Demux2/5 -> Bus Creator3/5  "Car Fr1 rvy"
  Demux2/6 -> Bus Creator3/6  "Car Fr1 rvz"
  Bus Creator3/1 -> Car.Fr1/1
  Kinetics/4 -> Demux2/1
  Car.Load/1 -> Kinetics/4
  Demux3/1 -> Bus Creator4/1  "car Susp FL GenInert2"
  Demux3/2 -> Bus Creator4/2  "car Susp FR GenInert2"
  Demux3/3 -> Bus Creator4/3  "car Susp FL GenFrc2"
  Demux3/4 -> Bus Creator4/4  "car Susp FR GenFrc2"
  Bus Creator4/1 -> WheelCarrier.Misc/1
  Bus Creator/1 -> Car.Trq_T2W/1
  Demux4/4 -> Bus Creator/4  "Car Trq_T2WRR"
  Demux4/3 -> Bus Creator/3  "Car Trq_T2WRL"
  Demux4/2 -> Bus Creator/2  "Car Trq_T2WFR"
  Demux4/1 -> Bus Creator/1  "Car Trq_T2WFL"
  TireFL.Out/1 -> Kinetics/5
  TireFR.Out/1 -> Kinetics/6
  TireRL.Out/1 -> Kinetics/7
  TireRR.Out/1 -> Kinetics/8
  FSpring/1 -> Kinetics/9
  FDamp/1 -> Kinetics/10
  FStabi/1 -> Kinetics/11
  Kinetics/6 -> Demux3/1
  Kinetics/5 -> Demux4/1

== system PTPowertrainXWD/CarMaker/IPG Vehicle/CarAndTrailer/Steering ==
  note: When replacing the entire steering system, be sure to add '-disablesteering' to the command line arguments in the CarMaker Model Configuration block.
  Sync_In : Inport
  VhclCtrl.Steering : Inport  Port=2
  Bus Creator1 : BusCreator  Inputs=16
  Bus Creator2 : BusCreator  Inputs=5
  Demux : Demux  Outputs=21
  Steering : S-Function  FunctionName=CM_Sfun  Parameters='Steering'
  Terminator : Terminator
  Sync_Out : Outport
  Steer.IF : Outport  Port=2
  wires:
  Demux/21 -> Bus Creator2/5  "Steering IF R Inert"
  Demux/20 -> Bus Creator2/4  "Steering IF R Frc"
  Demux/19 -> Bus Creator2/3  "Steering IF L Inert"
  Demux/18 -> Bus Creator2/2  "Steering IF L Frc"
  Demux/17 -> Bus Creator2/1  "Steering IF SteerByTrq"
  Demux/16 -> Bus Creator1/16  "Steering IF R iSteer2q"
  Demux/15 -> Bus Creator1/15  "Steering IF R qpp"
  Demux/14 -> Bus Creator1/14  "Steering IF R qp"
  Demux/13 -> Bus Creator1/13  "Steering IF R q"
  Demux/12 -> Bus Creator1/12  "Steering IF L iSteer2q"
  Demux/11 -> Bus Creator1/11  "Steering IF L qpp"
  Demux/10 -> Bus Creator1/10  "Steering IF L qp"
  Demux/9 -> Bus Creator1/9  "Steering IF L q"
  Demux/8 -> Bus Creator1/8  "Steering IF AssistTrqPin"
  Demux/7 -> Bus Creator1/7  "Steering IF AssistTrqCol"
  Demux/6 -> Bus Creator1/6  "Steering IF AssistFrc"
  Demux/5 -> Bus Creator1/5  "Steering IF TrqStatic"
  Demux/4 -> Bus Creator1/4  "Steering IF Trq"
  Demux/3 -> Bus Creator1/3  "Steering IF AngAcc"
  Demux/2 -> Bus Creator1/2  "Steering IF AngVel"
  Demux/1 -> Bus Creator1/1  "Steering IF Ang"
  Bus Creator1/1 -> Steer.IF/1
  Steering/2 -> Demux/1
  Bus Creator2/1 -> Terminator/1  "Steer IF (in)"
  VhclCtrl.Steering/1 -> Steering/2
  Steering/1 -> Sync_Out/1
  Sync_In/1 -> Steering/1

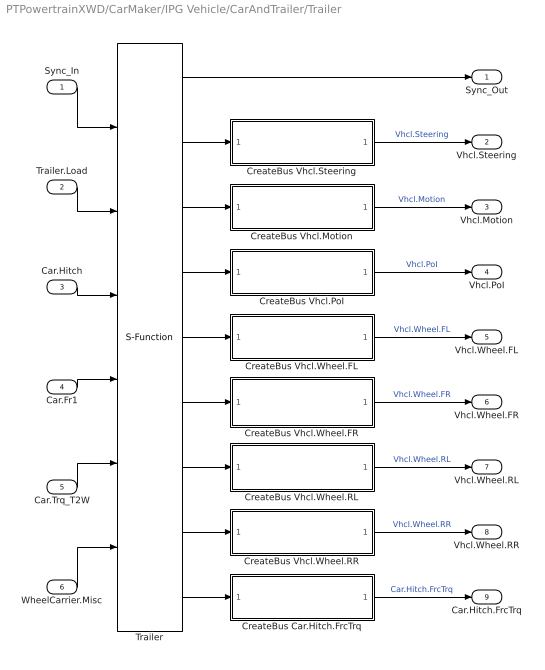
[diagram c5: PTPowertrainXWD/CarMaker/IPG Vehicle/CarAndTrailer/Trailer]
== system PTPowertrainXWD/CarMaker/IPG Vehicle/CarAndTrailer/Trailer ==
  Sync_In : Inport
  Trailer.Load : Inport  Port=2
  Car.Hitch : Inport  Port=3
  Car.Fr1 : Inport  Port=4
  Car.Trq_T2W : Inport  Port=5
  WheelCarrier.Misc : Inport  Port=6
  CreateBus Car.Hitch.FrcTrq : Subsystem
  CreateBus Vhcl.Motion : Subsystem
  CreateBus Vhcl.PoI : Subsystem
  CreateBus Vhcl.Steering : Subsystem
  CreateBus Vhcl.Wheel.FL : Subsystem
  CreateBus Vhcl.Wheel.FR : Subsystem
  CreateBus Vhcl.Wheel.RL : Subsystem
  CreateBus Vhcl.Wheel.RR : Subsystem
  Trailer : S-Function  FunctionName=CM_Sfun  Parameters='Trailer'
  Sync_Out : Outport
  Vhcl.Steering : Outport  Port=2
  Vhcl.Motion : Outport  Port=3
  Vhcl.PoI : Outport  Port=4
  Vhcl.Wheel.FL : Outport  Port=5
  Vhcl.Wheel.FR : Outport  Port=6
  Vhcl.Wheel.RL : Outport  Port=7
  Vhcl.Wheel.RR : Outport  Port=8
  Car.Hitch.FrcTrq : Outport  Port=9
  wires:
  Trailer/2 -> CreateBus Vhcl.Steering/1(In1)
  CreateBus Vhcl.Steering/1(Out1) -> Vhcl.Steering/1  "Vhcl.Steering"
  Trailer/3 -> CreateBus Vhcl.Motion/1(In1)
  Trailer/4 -> CreateBus Vhcl.PoI/1(In1)
  Trailer/5 -> CreateBus Vhcl.Wheel.FL/1(In1)
  Trailer/6 -> CreateBus Vhcl.Wheel.FR/1(In1)
  Trailer/7 -> CreateBus Vhcl.Wheel.RL/1(In1)
  Trailer/9 -> CreateBus Car.Hitch.FrcTrq/1(In1)
  Trailer/8 -> CreateBus Vhcl.Wheel.RR/1(In1)
  CreateBus Vhcl.Wheel.RR/1(Out1) -> Vhcl.Wheel.RR/1  "Vhcl.Wheel.RR"
  CreateBus Vhcl.Wheel.RL/1(Out1) -> Vhcl.Wheel.RL/1  "Vhcl.Wheel.RL"
  CreateBus Vhcl.Wheel.FR/1(Out1) -> Vhcl.Wheel.FR/1  "Vhcl.Wheel.FR"
  CreateBus Vhcl.Wheel.FL/1(Out1) -> Vhcl.Wheel.FL/1  "Vhcl.Wheel.FL"
  CreateBus Vhcl.PoI/1(Out1) -> Vhcl.PoI/1  "Vhcl.PoI"
  CreateBus Vhcl.Motion/1(Out1) -> Vhcl.Motion/1  "Vhcl.Motion"
  Car.Trq_T2W/1 -> Trailer/5
  WheelCarrier.Misc/1 -> Trailer/6
  CreateBus Car.Hitch.FrcTrq/1(Out1) -> Car.Hitch.FrcTrq/1  "Car.Hitch.FrcTrq"
  Car.Fr1/1 -> Trailer/4
  Car.Hitch/1 -> Trailer/3
  Trailer.Load/1 -> Trailer/2
  Trailer/1 -> Sync_Out/1
  Sync_In/1 -> Trailer/1

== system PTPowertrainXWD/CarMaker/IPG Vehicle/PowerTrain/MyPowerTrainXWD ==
  note: rotv
  note: Trq
  note: PowerTrain.Motor.Mot.TrqMap: 0 300.0 700 300.0 1400 150.0 2100 100.0 3000 75.0 8000 20.0
  PT.WFL.rotv : Inport
  PT.WFR.rotv : Inport  Port=2
  Gas : Inport  Port=3
  iDiff_mean : Inport  Port=4
  " " : Gain  Gain=1/2
  "  " : Gain  Gain=1/2
  "   " : Product
  "    " : Product
  "  1" : Gain  Gain=-1
  1-D Lookup Table : Lookup_n-D  NumberOfTableDimensions=1  BreakpointsForDimension1=[0,700,1400,2100,3000,8000]  Table=[300,300,150,100,75,20]  InternalRulePriority=Speed  RndMeth=Simplest
  Abs : Abs
  Product1 : Product
  Sum : Sum  Inputs=|++
  PT.WFL.Trq_Drive : Outport
  PT.WFR.Trq_Drive : Outport  Port=2
  PT.WFL.Trq_Supp2WC : Outport  Port=3
  PT.WFR.Trq_Supp2WC : Outport  Port=4
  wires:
  "  1"/1 -> PT.WFL.Trq_Supp2WC/1, PT.WFR.Trq_Supp2WC/1
  "   "/1 -> PT.WFL.Trq_Drive/1, "  1"/1, PT.WFR.Trq_Drive/1
  "  "/1 -> "   "/2
  Product1/1 -> "  "/1
  Gas/1 -> Product1/2
  1-D Lookup Table/1 -> Product1/1
  "    "/1 -> Abs/1
  iDiff_mean/1 -> "   "/1, "    "/1
  " "/1 -> "    "/2
  Sum/1 -> " "/1
  PT.WFR.rotv/1 -> Sum/2
  PT.WFL.rotv/1 -> Sum/1
  Abs/1 -> 1-D Lookup Table/1

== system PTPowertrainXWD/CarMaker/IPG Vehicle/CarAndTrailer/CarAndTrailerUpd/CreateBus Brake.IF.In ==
  In : Inport
  BusCreator : BusCreator  Inputs=9
  Demux : Demux  Outputs=9
  Out : Outport
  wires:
  Demux/9 -> BusCreator/9  "Brake IF Trq_Reg RR"
  Demux/8 -> BusCreator/8  "Brake IF Trq_Reg RL"
  Demux/7 -> BusCreator/7  "Brake IF Trq_Reg FR"
  Demux/6 -> BusCreator/6  "Brake IF Trq_Reg FL"
  Demux/5 -> BusCreator/5  "Brake IF Trq_Reg_max RR"
  Demux/4 -> BusCreator/4  "Brake IF Trq_Reg_max RL"
  Demux/3 -> BusCreator/3  "Brake IF Trq_Reg_max FR"
  Demux/2 -> BusCreator/2  "Brake IF Trq_Reg_max FL"
  Demux/1 -> BusCreator/1  "Brake IF T_env"
  BusCreator/1 -> Out/1
  In/1 -> Demux/1

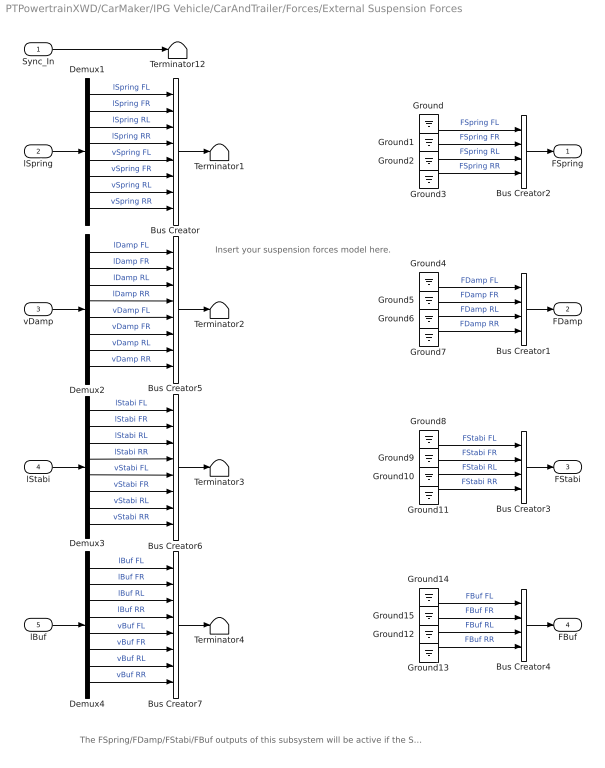
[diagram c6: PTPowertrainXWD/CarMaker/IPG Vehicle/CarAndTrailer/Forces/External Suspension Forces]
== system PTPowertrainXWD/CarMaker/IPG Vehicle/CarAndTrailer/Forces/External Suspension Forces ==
  note: The FSpring/FDamp/FStabi/FBuf outputs of this subsystem will be active if the SuspExtFrcs.Kind entry in the vehicle parameter file is either not present or is empty or has the value "CM4SL".
  note: Insert your suspension forces model here.
  Sync_In : Inport
  lSpring : Inport  Port=2
  vDamp : Inport  Port=3
  lStabi : Inport  Port=4
  lBuf : Inport  Port=5
  Bus Creator{,5..7} (4 alike) : BusCreator  Inputs=8
  Bus Creator{1..4} (4 alike) : BusCreator
  Demux{1..4} (4 alike) : Demux  Outputs=8
  Ground{,1..15} (16 alike) : Ground
  Terminator{1..4,12} (5 alike) : Terminator
  FSpring : Outport
  FDamp : Outport  Port=2
  FStabi : Outport  Port=3
  FBuf : Outport  Port=4
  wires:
  Bus Creator7/1 -> Terminator4/1
  Bus Creator6/1 -> Terminator3/1
  Bus Creator5/1 -> Terminator2/1
  Bus Creator/1 -> Terminator1/1
  Demux4/8 -> Bus Creator7/8  "vBuf RR"
  Demux4/7 -> Bus Creator7/7  "vBuf RL"
  Demux4/6 -> Bus Creator7/6  "vBuf FR"
  Demux4/5 -> Bus Creator7/5  "vBuf FL"
  Demux3/8 -> Bus Creator6/8  "vStabi RR"
  Demux3/7 -> Bus Creator6/7  "vStabi RL"
  Demux3/6 -> Bus Creator6/6  "vStabi FR"
  Demux3/5 -> Bus Creator6/5  "vStabi FL"
  Demux2/8 -> Bus Creator5/8  "vDamp RR"
  Demux2/7 -> Bus Creator5/7  "vDamp RL"
  Demux2/6 -> Bus Creator5/6  "vDamp FR"
  Demux2/5 -> Bus Creator5/5  "vDamp FL"
  Demux1/8 -> Bus Creator/8  "vSpring RR"
  Demux1/7 -> Bus Creator/7  "vSpring RL"
  Demux1/6 -> Bus Creator/6  "vSpring FR"
  Demux1/5 -> Bus Creator/5  "vSpring FL"
  Demux2/4 -> Bus Creator5/4  "lDamp RR"
  Demux2/3 -> Bus Creator5/3  "lDamp RL"
  Demux2/2 -> Bus Creator5/2  "lDamp FR"
  Demux2/1 -> Bus Creator5/1  "lDamp FL"
  Demux1/4 -> Bus Creator/4  "lSpring RR"
  Demux1/3 -> Bus Creator/3  "lSpring RL"
  Demux1/2 -> Bus Creator/2  "lSpring FR"
  Demux1/1 -> Bus Creator/1  "lSpring FL"
  Demux3/4 -> Bus Creator6/4  "lStabi RR"
  Demux3/3 -> Bus Creator6/3  "lStabi RL"
  Demux3/2 -> Bus Creator6/2  "lStabi FR"
  Demux3/1 -> Bus Creator6/1  "lStabi FL"
  lStabi/1 -> Demux3/1
  vDamp/1 -> Demux2/1
  lSpring/1 -> Demux1/1
  Demux4/4 -> Bus Creator7/4  "lBuf RR"
  Demux4/3 -> Bus Creator7/3  "lBuf RL"
  Demux4/2 -> Bus Creator7/2  "lBuf FR"
  Demux4/1 -> Bus Creator7/1  "lBuf FL"
  lBuf/1 -> Demux4/1
  Ground14/1 -> Bus Creator4/1  "FBuf FL"
  Ground15/1 -> Bus Creator4/2  "FBuf FR"
  Ground12/1 -> Bus Creator4/3  "FBuf RL"
  Ground13/1 -> Bus Creator4/4  "FBuf RR"
  Bus Creator4/1 -> FBuf/1
  Sync_In/1 -> Terminator12/1
  Bus Creator2/1 -> FSpring/1
  Ground/1 -> Bus Creator2/1  "FSpring FL"
  Ground1/1 -> Bus Creator2/2  "FSpring FR"
  Ground2/1 -> Bus Creator2/3  "FSpring RL"
  Ground3/1 -> Bus Creator2/4  "FSpring RR"
  Ground4/1 -> Bus Creator1/1  "FDamp FL"
  Ground5/1 -> Bus Creator1/2  "FDamp FR"
  Ground6/1 -> Bus Creator1/3  "FDamp RL"
  Ground7/1 -> Bus Creator1/4  "FDamp RR"
  Bus Creator1/1 -> FDamp/1
  Ground8/1 -> Bus Creator3/1  "FStabi FL"
  Ground9/1 -> Bus Creator3/2  "FStabi FR"
  Ground10/1 -> Bus Creator3/3  "FStabi RL"
  Ground11/1 -> Bus Creator3/4  "FStabi RR"
  Bus Creator3/1 -> FStabi/1

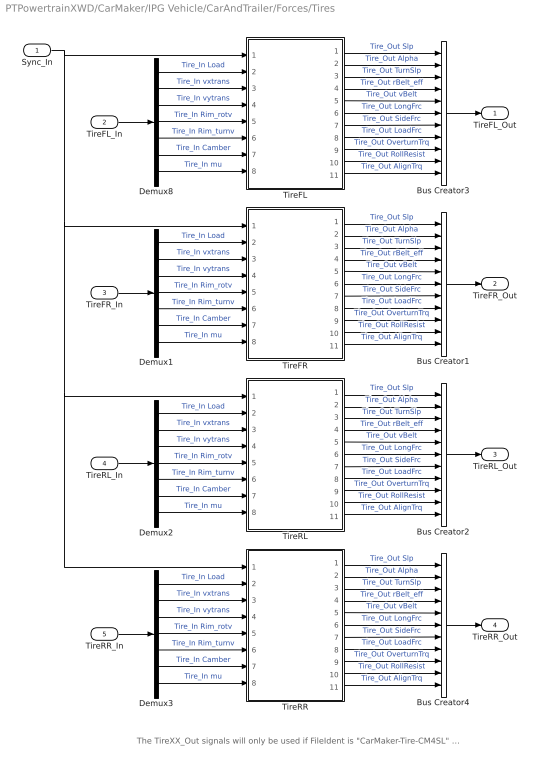
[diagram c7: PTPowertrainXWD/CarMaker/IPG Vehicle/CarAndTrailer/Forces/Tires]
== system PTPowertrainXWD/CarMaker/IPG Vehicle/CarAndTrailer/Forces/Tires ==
  note: The TireXX_Out signals will only be used if FileIdent is "CarMaker-Tire-CM4SL" in the tire parameter file! An example parameter file can be found in Data/Tire/DT_CM4SL_UserTire.
  Sync_In : Inport
  TireFL_In : Inport  Port=2
  TireFR_In : Inport  Port=3
  TireRL_In : Inport  Port=4
  TireRR_In : Inport  Port=5
  Bus Creator{1..4} (4 alike) : BusCreator  Inputs=11
  Demux{1..3,8} (4 alike) : Demux  Outputs=7
  TireFL : Subsystem
  TireFR : Subsystem
  TireRL : Subsystem
  TireRR : Subsystem
  TireFL_Out : Outport
  TireFR_Out : Outport  Port=2
  TireRL_Out : Outport  Port=3
  TireRR_Out : Outport  Port=4
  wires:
  Sync_In/1 -> TireRR/1(Sync_In), TireRL/1(Sync_In), TireFR/1(Sync_In), TireFL/1(Sync_In)
  Bus Creator4/1 -> TireRR_Out/1
  Bus Creator2/1 -> TireRL_Out/1
  Bus Creator1/1 -> TireFR_Out/1
  Demux3/5 -> TireRR/6(Rim_turnv)  "Tire_In Rim_turnv"
  Demux3/4 -> TireRR/5(Rim_rotv)  "Tire_In Rim_rotv"
  Demux3/1 -> TireRR/2(Load)  "Tire_In Load"
  Demux3/7 -> TireRR/8(muRoad)  "Tire_In mu"
  Demux3/6 -> TireRR/7(InclinAngle)  "Tire_In Camber"
  Demux3/2 -> TireRR/3(vxtrans)  "Tire_In vxtrans"
  Demux3/3 -> TireRR/4(vytrans)  "Tire_In vytrans"
  TireRR/11(AlignTrq) -> Bus Creator4/11  "Tire_Out AlignTrq"
  TireRR/10(RollResist) -> Bus Creator4/10  "Tire_Out RollResist"
  TireRR/9(OverturnTrq) -> Bus Creator4/9  "Tire_Out OverturnTrq"
  TireRR/8(LoadFrc) -> Bus Creator4/8  "Tire_Out LoadFrc"
  TireRR/7(SideFrc) -> Bus Creator4/7  "Tire_Out SideFrc"
  TireRR/6(LongFrc) -> Bus Creator4/6  "Tire_Out LongFrc"
  TireRR/5(vBelt) -> Bus Creator4/5  "Tire_Out vBelt"
  TireRR/4(rBelt_eff) -> Bus Creator4/4  "Tire_Out rBelt_eff"
  TireRR/3(TurnSlp) -> Bus Creator4/3  "Tire_Out TurnSlp"
  TireRR/1(Slp) -> Bus Creator4/1  "Tire_Out Slp"
  TireRR/2(Alpha) -> Bus Creator4/2  "Tire_Out Alpha"
  Demux2/5 -> TireRL/6(Rim_turnv)  "Tire_In Rim_turnv"
  Demux2/4 -> TireRL/5(Rim_rotv)  "Tire_In Rim_rotv"
  Demux2/1 -> TireRL/2(Load)  "Tire_In Load"
  Demux2/7 -> TireRL/8(muRoad)  "Tire_In mu"
  Demux2/6 -> TireRL/7(InclinAngle)  "Tire_In Camber"
  Demux2/2 -> TireRL/3(vxtrans)  "Tire_In vxtrans"
  Demux2/3 -> TireRL/4(vytrans)  "Tire_In vytrans"
  TireRL/11(AlignTrq) -> Bus Creator2/11  "Tire_Out AlignTrq"
  TireRL/10(RollResist) -> Bus Creator2/10  "Tire_Out RollResist"
  TireRL/9(OverturnTrq) -> Bus Creator2/9  "Tire_Out OverturnTrq"
  TireRL/8(LoadFrc) -> Bus Creator2/8  "Tire_Out LoadFrc"
  TireRL/7(SideFrc) -> Bus Creator2/7  "Tire_Out SideFrc"
  TireRL/6(LongFrc) -> Bus Creator2/6  "Tire_Out LongFrc"
  TireRL/5(vBelt) -> Bus Creator2/5  "Tire_Out vBelt"
  TireRL/4(rBelt_eff) -> Bus Creator2/4  "Tire_Out rBelt_eff"
  TireRL/3(TurnSlp) -> Bus Creator2/3  "Tire_Out TurnSlp"
  TireRL/1(Slp) -> Bus Creator2/1  "Tire_Out Slp"
  TireRL/2(Alpha) -> Bus Creator2/2  "Tire_Out Alpha"
  Demux1/5 -> TireFR/6(Rim_turnv)  "Tire_In Rim_turnv"
  Demux1/4 -> TireFR/5(Rim_rotv)  "Tire_In Rim_rotv"
  Demux1/1 -> TireFR/2(Load)  "Tire_In Load"
  Demux1/7 -> TireFR/8(muRoad)  "Tire_In mu"
  Demux1/6 -> TireFR/7(InclinAngle)  "Tire_In Camber"
  Demux1/2 -> TireFR/3(vxtrans)  "Tire_In vxtrans"
  Demux1/3 -> TireFR/4(vytrans)  "Tire_In vytrans"
  TireFR/11(AlignTrq) -> Bus Creator1/11  "Tire_Out AlignTrq"
  TireFR/10(RollResist) -> Bus Creator1/10  "Tire_Out RollResist"
  TireFR/9(OverturnTrq) -> Bus Creator1/9  "Tire_Out OverturnTrq"
  TireFR/8(LoadFrc) -> Bus Creator1/8  "Tire_Out LoadFrc"
  TireFR/7(SideFrc) -> Bus Creator1/7  "Tire_Out SideFrc"
  TireFR/6(LongFrc) -> Bus Creator1/6  "Tire_Out LongFrc"
  TireFR/5(vBelt) -> Bus Creator1/5  "Tire_Out vBelt"
  TireFR/4(rBelt_eff) -> Bus Creator1/4  "Tire_Out rBelt_eff"
  TireFR/3(TurnSlp) -> Bus Creator1/3  "Tire_Out TurnSlp"
  TireFR/1(Slp) -> Bus Creator1/1  "Tire_Out Slp"
  TireFR/2(Alpha) -> Bus Creator1/2  "Tire_Out Alpha"
  Demux8/5 -> TireFL/6(Rim_turnv)  "Tire_In Rim_turnv"
  Demux8/4 -> TireFL/5(Rim_rotv)  "Tire_In Rim_rotv"
  TireFL_In/1 -> Demux8/1
  Demux8/1 -> TireFL/2(Load)  "Tire_In Load"
  Demux8/7 -> TireFL/8(muRoad)  "Tire_In mu"
  Demux8/6 -> TireFL/7(InclinAngle)  "Tire_In Camber"
  Demux8/2 -> TireFL/3(vxtrans)  "Tire_In vxtrans"
  Demux8/3 -> TireFL/4(vytrans)  "Tire_In vytrans"
  TireFL/11(AlignTrq) -> Bus Creator3/11  "Tire_Out AlignTrq"
  TireFL/10(RollResist) -> Bus Creator3/10  "Tire_Out RollResist"
  TireFL/9(OverturnTrq) -> Bus Creator3/9  "Tire_Out OverturnTrq"
  TireFL/8(LoadFrc) -> Bus Creator3/8  "Tire_Out LoadFrc"
  TireFL/7(SideFrc) -> Bus Creator3/7  "Tire_Out SideFrc"
  TireFL/6(LongFrc) -> Bus Creator3/6  "Tire_Out LongFrc"
  TireFL/5(vBelt) -> Bus Creator3/5  "Tire_Out vBelt"
  TireFL/4(rBelt_eff) -> Bus Creator3/4  "Tire_Out rBelt_eff"
  TireFL/3(TurnSlp) -> Bus Creator3/3  "Tire_Out TurnSlp"
  TireFL/1(Slp) -> Bus Creator3/1  "Tire_Out Slp"
  TireFL/2(Alpha) -> Bus Creator3/2  "Tire_Out Alpha"
  Bus Creator3/1 -> TireFL_Out/1
  TireFR_In/1 -> Demux1/1
  TireRL_In/1 -> Demux2/1
  TireRR_In/1 -> Demux3/1

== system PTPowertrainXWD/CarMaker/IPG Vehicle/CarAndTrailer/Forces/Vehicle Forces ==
  Sync_In : Inport
  Bus Creator1 : BusCreator  Inputs=12
  Bus Creator8 : BusCreator  Inputs=16
  BusCreator1 : BusCreator
  BusCreator2 : BusCreator  Inputs=9
  Demux : Demux  Outputs=16
  Demux1 : Demux  Outputs=12
  Demux2 : Demux  Outputs=13
  Forces : S-Function  FunctionName=CM_Sfun  Parameters='Forces'
  Terminator : Terminator
  Sync_Out : Outport
  Car.Virtual : Outport  Port=2
  Car.Aero : Outport  Port=3
  Car.Load : Outport  Port=4
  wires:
  BusCreator1/1 -> Terminator/1  "Aero IF (in)"
  Demux2/13 -> BusCreator2/9  "car Aero Trq_1 z"
  Demux2/12 -> BusCreator2/8  "car Aero Trq_1 y"
  Demux2/11 -> BusCreator2/7  "car Aero Trq_1 x"
  Demux2/10 -> BusCreator2/6  "car Aero Frc_1 z"
  Demux2/9 -> BusCreator2/5  "car Aero Frc_1 y"
  Demux2/8 -> BusCreator2/4  "car Aero Frc_1 x"
  Demux2/7 -> BusCreator2/3  "car Aero PoA_1 z"
  Demux2/6 -> BusCreator2/2  "car Aero PoA_1 y"
  Demux2/5 -> BusCreator2/1  "car Aero PoA_1 x"
  Demux2/4 -> BusCreator1/4  "car Aero tau_1"
  Demux2/3 -> BusCreator1/3  "car Aero ApproachVel_1 z"
  Demux2/2 -> BusCreator1/2  "car Aero ApproachVel_1 y"
  Demux2/1 -> BusCreator1/1  "car Aero ApproachVel_1 x"
  Demux/16 -> Bus Creator8/16  "Car Load_3 tz"
  Demux/15 -> Bus Creator8/15  "Car Load_3 ty"
  Demux/14 -> Bus Creator8/14  "Car Load_3 tx"
  Demux/13 -> Bus Creator8/13  "Car Load_3 mass"
  Demux1/12 -> Bus Creator1/12  "Car Virtual Trq_0 z"
  Demux1/11 -> Bus Creator1/11  "Car Virtual Trq_0 y"
  Demux1/10 -> Bus Creator1/10  "Car Virtual Trq_0 x"
  Demux1/9 -> Bus Creator1/9  "Car Virtual Trq_1 z"
  Demux1/8 -> Bus Creator1/8  "Car Virtual Trq_1 y"
  Demux1/7 -> Bus Creator1/7  "Car Virtual Trq_1 x"
  Demux1/6 -> Bus Creator1/6  "Car Virtual Frc_0 z"
  Demux1/5 -> Bus Creator1/5  "Car Virtual Frc_0 y"
  Demux1/4 -> Bus Creator1/4  "Car Virtual Frc_0 x"
  Sync_In/1 -> Forces/1
  Forces/1 -> Sync_Out/1
  BusCreator2/1 -> Car.Aero/1
  Demux1/1 -> Bus Creator1/1  "Car Virtual Frc_1 x"
  Demux1/2 -> Bus Creator1/2  "Car Virtual Frc_1 y"
  Demux1/3 -> Bus Creator1/3  "Car Virtual Frc_1 z"
  Forces/3 -> Demux2/1
  Forces/2 -> Demux1/1
  Bus Creator1/1 -> Car.Virtual/1
  Bus Creator8/1 -> Car.Load/1
  Demux/1 -> Bus Creator8/1  "Car Load_0 mass"
  Demux/2 -> Bus Creator8/2  "Car Load_0 tx"
  Demux/3 -> Bus Creator8/3  "Car Load_0 ty"
  Demux/4 -> Bus Creator8/4  "Car Load_0 tz"
  Demux/5 -> Bus Creator8/5  "Car Load_1 mass"
  Demux/6 -> Bus Creator8/6  "Car Load_1 tx"
  Demux/7 -> Bus Creator8/7  "Car Load_1 ty"
  Demux/8 -> Bus Creator8/8  "Car Load_1 tz"
  Demux/9 -> Bus Creator8/9  "Car Load_2 mass"
  Demux/10 -> Bus Creator8/10  "Car Load_2 tx"
  Demux/11 -> Bus Creator8/11  "Car Load_2 ty"
  Demux/12 -> Bus Creator8/12  "Car Load_2 tz"
  Forces/4 -> Demux/1

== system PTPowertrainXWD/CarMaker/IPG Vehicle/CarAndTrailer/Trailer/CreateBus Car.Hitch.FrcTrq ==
  In1 : Inport
  Bus Creator7 : BusCreator  Inputs=6
  Demux7 : Demux  Outputs=6
  Out1 : Outport
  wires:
  In1/1 -> Demux7/1
  Bus Creator7/1 -> Out1/1
  Demux7/6 -> Bus Creator7/6  "Car Hitch Trq2Car z"
  Demux7/5 -> Bus Creator7/5  "Car Hitch Trq2Car y"
  Demux7/4 -> Bus Creator7/4  "Car Hitch Trq2Car x"
  Demux7/3 -> Bus Creator7/3  "Car Hitch Frc2Car z"
  Demux7/2 -> Bus Creator7/2  "Car Hitch Frc2Car y"
  Demux7/1 -> Bus Creator7/1  "Car Hitch Frc2Car x"

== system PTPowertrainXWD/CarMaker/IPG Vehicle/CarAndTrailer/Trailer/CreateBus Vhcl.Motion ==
  In1 : Inport
  BusCreator : BusCreator  Inputs=15
  Demux : Demux  Outputs=15
  Out1 : Outport
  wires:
  Demux/15 -> BusCreator/15  "Vhcl YawAcc"
  Demux/14 -> BusCreator/14  "Vhcl YawVel"
  Demux/13 -> BusCreator/13  "Vhcl Yaw"
  Demux/12 -> BusCreator/12  "Vhcl PitchAcc"
  Demux/11 -> BusCreator/11  "Vhcl PitchVel"
  Demux/10 -> BusCreator/10  "Vhcl Pitch"
  Demux/9 -> BusCreator/9  "Vhcl RollAcc"
  Demux/8 -> BusCreator/8  "Vhcl RollVel"
  Demux/7 -> BusCreator/7  "Vhcl Roll"
  Demux/6 -> BusCreator/6  "Vhcl Hitch_Pos z"
  Demux/5 -> BusCreator/5  "Vhcl Hitch_Pos y"
  Demux/4 -> BusCreator/4  "Vhcl Hitch_Pos x"
  Demux/3 -> BusCreator/3  "Vhcl sRoad"
  Demux/2 -> BusCreator/2  "Vhcl Distance"
  Demux/1 -> BusCreator/1  "Vhcl v"
  In1/1 -> Demux/1
  BusCreator/1 -> Out1/1

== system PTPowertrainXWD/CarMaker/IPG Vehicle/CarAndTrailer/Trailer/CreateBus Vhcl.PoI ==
  In1 : Inport
  Bus Creator3 : BusCreator  Inputs=18
  Demux3 : Demux  Outputs=18
  Out1 : Outport
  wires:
  Demux3/18 -> Bus Creator3/18  "Vhcl PoI_GCS Elev"
  Demux3/17 -> Bus Creator3/17  "Vhcl PoI_GCS Lat"
  Demux3/16 -> Bus Creator3/16  "Vhcl PoI_GCS Long"
  Demux3/15 -> Bus Creator3/15  "Vhcl PoI_Acc_1 z"
  Demux3/14 -> Bus Creator3/14  "Vhcl PoI_Acc_1 y"
  Demux3/13 -> Bus Creator3/13  "Vhcl PoI_Acc_1 x"
  Demux3/12 -> Bus Creator3/12  "Vhcl PoI_Vel_1 z"
  Demux3/11 -> Bus Creator3/11  "Vhcl PoI_Vel_1 y"
  Demux3/10 -> Bus Creator3/10  "Vhcl PoI_Vel_1 x"
  Demux3/9 -> Bus Creator3/9  "Vhcl PoI_Acc z"
  Demux3/8 -> Bus Creator3/8  "Vhcl PoI_Acc y"
  Demux3/7 -> Bus Creator3/7  "Vhcl PoI_Acc x"
  Demux3/6 -> Bus Creator3/6  "Vhcl PoI_Vel z"
  Demux3/5 -> Bus Creator3/5  "Vhcl PoI_Vel y"
  Demux3/4 -> Bus Creator3/4  "Vhcl PoI_Vel x"
  Demux3/3 -> Bus Creator3/3  "Vhcl PoI_Pos z"
  Demux3/2 -> Bus Creator3/2  "Vhcl PoI_Pos y"
  In1/1 -> Demux3/1
  Bus Creator3/1 -> Out1/1
  Demux3/1 -> Bus Creator3/1  "Vhcl PoI_Pos x"

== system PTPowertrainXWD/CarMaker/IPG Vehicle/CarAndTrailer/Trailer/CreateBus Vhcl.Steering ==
  In1 : Inport
  Bus Creator3 : BusCreator
  Demux : Demux
  Out1 : Outport
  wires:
  Bus Creator3/1 -> Out1/1
  Demux/1 -> Bus Creator3/1  "Vhcl Steering Ang"
  Demux/3 -> Bus Creator3/3  "Vhcl Steering AngAcc"
  Demux/2 -> Bus Creator3/2  "Vhcl Steering AngVel"
  Demux/4 -> Bus Creator3/4  "Vhcl Steering Trq"
  In1/1 -> Demux/1
